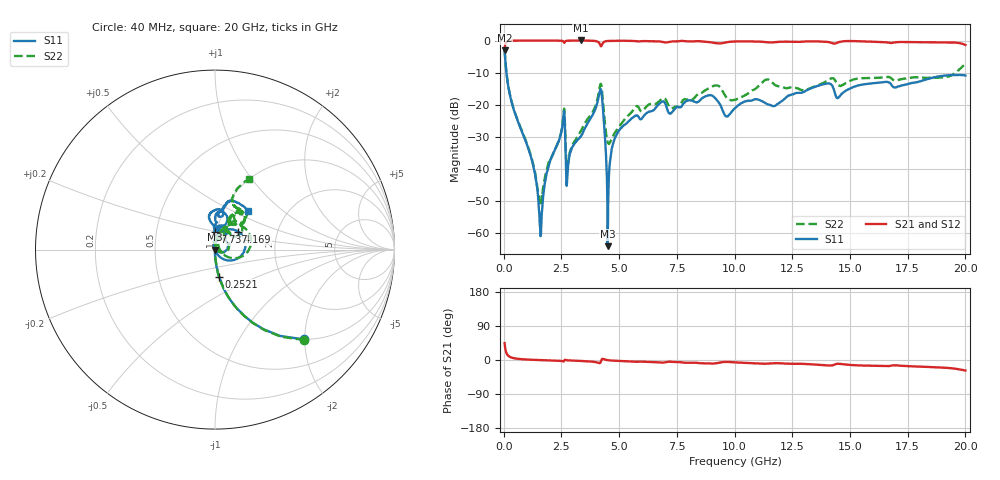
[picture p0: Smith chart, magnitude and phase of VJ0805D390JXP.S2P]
! VJ0805D390JXP
! DATE 10/29/2021  12:46
! CAPACITORS MOUNTED IN SERIES ON 25 MIL THICK MICROSTRIP SUBSTRATE
# GHz  S  MA  R  50.00
!  FREQ  S11M  S11A  S21M  S21A  S12M  S12A  S22M  S22A
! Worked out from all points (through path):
!   1601 points, 40 MHz to 20 GHz, reference 50 ohm
!   highest |S21| = 0.03 dB at 3.346 GHz (marker M1); lowest = -3.0 dB at 40 MHz (marker M2)
!   group delay of S21, straight-line fit = 3.23 ps
!   lowest |S11| = -64.2 dB at 4.506 GHz (marker M3), VSWR 1.00, Z = 50 - j0.0479 ohm
!   |S11| at or under -10 dB: 118.8 MHz to end of sweep
!   |S22| runs from -51.6 to -3.0 dB; largest |S21 - S12| = 0.0087
!   S11 on the Smith chart (normalised r, x): 40 MHz: 1.00, -1.98; 252.1 MHz: 1.00, -0.31; 4.169 GHz: 1.27, +0.26; 7.737 GHz: 0.98, +0.19; 20 GHz: 1.29, +0.61
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0.04  0.7042 -45.3  0.7061 44.6  0.704 44.6  0.7085 -45.4
0.252075  0.1522 -81.5  0.9877 8.6  0.9878 8.5  0.1538 -81.2
1.250075  0.01231 -93.9  0.9989 0.6  0.999 0.5  0.01302 -80.8
1.5869  0.001119 -160.3  0.999 -0.2  0.9994 -0.3  0.002623 -2.7
1.923725  0.009994 89.7  0.9979 -0.8  0.9987 -0.9  0.0114 72.7
2.547475  0.04768 79.3  0.989 -3.1  0.9896 -3.1  0.05004 72.3
2.7845  0.0105 84.9  0.9957 -0.9  0.9964 -1.0  0.01251 58.3
3.345875  0.03191 96.6  1.004 -2.5  1.004 -2.6  0.039 89.8
3.370825  0.03301 97.9  1.003 -2.6  1.004 -2.7  0.04054 90.4
4.169225  0.1644 37.3  0.871 -8.1  0.8721 -8.2  0.1958 43.6
4.293975  0.09201 -40.9  0.9109 3.0  0.9115 2.9  0.1187 -23.9
4.50605  0.0006146 -128.8  0.9861 -0.4  0.9872 -0.5  0.02575 5.5
4.7306  0.02397 99.1  0.9929 -1.8  0.9942 -1.9  0.03168 56.5
5.00505  0.03974 91.6  0.9952 -2.8  0.9953 -2.9  0.04528 70.7
6.70165  0.09915 78.5  0.9721 -6.4  0.9724 -6.5  0.1096 63.6
7.737075  0.09734 91.0  0.9878 -6.5  0.9883 -6.7  0.1134 67.0
9.19665  0.122 57.3  0.9115 -8.6  0.9118 -8.8  0.1995 47.1
10.02  0.08756 90.2  0.9699 -6.2  0.9697 -6.4  0.1187 52.3
11.39225  0.1029 74.1  0.9408 -9.8  0.9415 -10.1  0.2469 54.3
13.35083  0.1814 89.2  0.9727 -11.6  0.9734 -11.8  0.1848 63.5
16.68165  0.2223 80.2  0.9254 -16.0  0.9261 -16.2  0.2692 49.2
20  0.2842 49.7  0.8535 -27.8  0.8535 -28.2  0.4371 64.1
